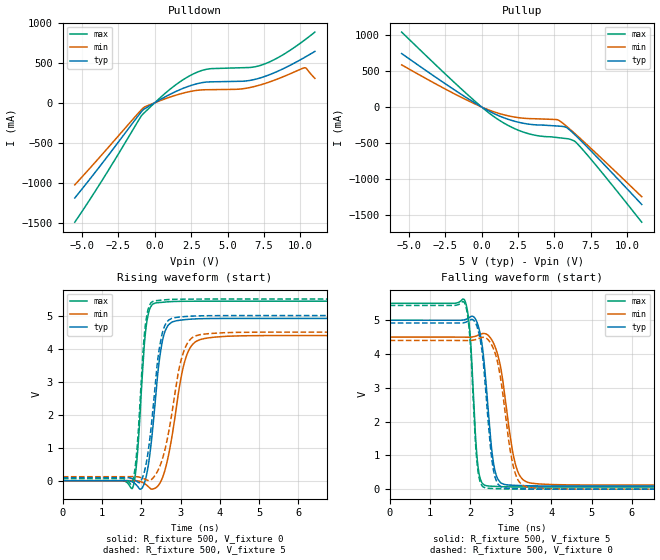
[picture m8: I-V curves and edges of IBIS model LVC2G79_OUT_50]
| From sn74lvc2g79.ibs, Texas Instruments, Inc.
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[Model]   LVC2G79_OUT_50
Model_type  Output
Vref =   0
Rref =   500
Cref =   50p
Vmeas =   2.5
| variable   typ   min   max
C_comp   8.95pF   5.46pF   12.36pF
| C_pullup   9.69pF   5.46pF   12.36pF
| C_pulldown   8.21pF   6.20pF   11.61pF
[Temperature Range]   40   100   -40
| Ambient temperature   25   85   -40
[Voltage range]   5   4.5   5.5
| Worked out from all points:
|   slope of the pulldown table from 0 to 0.75 V, typ, clamps not added: 9.73 ohm
|   slope of the pullup table from 0 to 0.75 V, typ, clamps not added: 9.16 ohm
|   rising waveform, R_fixture 500, V_fixture 0: 20-80 % time 258ps typ, 373ps min, 175ps max; typ from 0 V to 4.91 V
|   falling waveform, R_fixture 500, V_fixture 5: 20-80 % time 221ps typ, 319ps min, 148ps max; typ from 5 V to 0.091 V
|   rising waveform, R_fixture 500, V_fixture 5: 20-80 % time 265ps typ, 395ps min, 175ps max; typ from 0.091 V to 5 V
|   falling waveform, R_fixture 500, V_fixture 0: 20-80 % time 218ps typ, 313ps min, 147ps max; typ from 4.92 V to 0 V
[Pulldown]
| LVC2G79_OUT_50
|   Voltage   I(typ)   I(min)   I(max)
-5.5V     -1.19A     -1.026A    -1.493A
-3.615V   -756.5mA   -644.9mA   -968mA
-860mV    -99.61mA   -76.72mA   -149.6mA
1.145V    114mA      76.72mA    182.7mA
2.335V    206.5mA    136.8mA    330.4mA
3.39V     254.8mA    162mA      411mA
5.9V      268mA      171.6mA    436.9mA
6.79V     288.1mA    200.2mA    446mA
7.59V     330.6mA    241.7mA    487.6mA
8.82V     424.5mA    324.7mA    600.5mA
10.29V    565.4mA    436.9mA    781.9mA
11V       641.1mA    304.6mA    882.6mA
[Pullup]
| LVC2G79_OUT_50
|   Voltage   I(typ)   I(min)   I(max)
-5.5V     745.2mA    587.5mA    1.044A
-1.18V    147.6mA    112.6mA    211.7mA
1.04V     -109.2mA   -79.97mA   -161.6mA
2.045V    -185.4mA   -131.8mA   -280mA
3.05V     -232.7mA   -158.7mA   -361.3mA
3.945V    -250.5mA   -165.3mA   -402.5mA
5.295V    -265.8mA   -184.8mA   -427.6mA
5.83V     -285.1mA   -267.5mA   -440mA
6.335V    -372.8mA   -357.2mA   -470.5mA
6.54V     -412.8mA   -394.7mA   -503.8mA
8.12V     -739mA     -692.4mA   -876.8mA
11V       -1.358A    -1.25A     -1.605A
[Ramp]
| LVC2G79_OUT_50
| variable   typ   min   max
dV/dt_r   3.10/2.76E-10   2.79/4.06E-10   3.41/1.90E-10
dV/dt_f   3.02/2.32E-10   2.69/3.36E-10   3.34/1.55E-10
R_load = 500
[Rising Waveform]
| LVC2G79_OUT_50
R_fixture =   500
C_fixture =   0
L_fixture =   0
V_fixture =   0
V_fixture_min = 0
V_fixture_max = 0
|   Time   V(typ)   V(min)   V(max)
0s        185.3pV    4.77nV     2.097nV
1.78ns    -40.47mV   4.267mV    -217.7mV
1.895ns   -154.8mV   -1.104mV   706.8mV
2.125ns   123.6mV    -121.8mV   4.669V
2.375ns   2.639V     -210.8mV   5.385V
2.52ns    4.114V     31.46mV    5.4V
2.67ns    4.68V      634.9mV    5.416V
3.115ns   4.877V     3.642V     5.433V
3.605ns   4.908V     4.304V     5.435V
22.5ns    4.914V     4.397V     5.435V
[Falling Waveform]
| LVC2G79_OUT_50
R_fixture =   500
C_fixture =   0
L_fixture =   0
V_fixture =   5
V_fixture_min = 4.5
V_fixture_max = 5.5
|   Time   V(typ)   V(min)   V(max)
0s        5V         4.5V       5.5V
1.86ns    5.015V     4.498V     5.584V
1.99ns    5.093V     4.498V     4.616V
2.185ns   4.86V      4.553V     697.9mV
2.405ns   2.875V     4.583V     99.76mV
2.54ns    1.041V     4.396V     86.95mV
2.67ns    318.2mV    4.002V     78.52mV
3.105ns   113.5mV    781.3mV    66.24mV
3.5ns     99.06mV    178.3mV    63.91mV
22.5ns    91.35mV    120.7mV    62.83mV
[Rising Waveform]
| LVC2G79_OUT_50
R_fixture =   500
C_fixture =   0
L_fixture =   0
V_fixture =   5
V_fixture_min = 4.5
V_fixture_max = 5.5
|   Time   V(typ)   V(min)   V(max)
0s        91.33mV    120.7mV    62.82mV
1.765ns   63.77mV    124.3mV    -75.71mV
1.885ns   -17.21mV   121.4mV    880.2mV
2.105ns   400.1mV    39.54mV    4.708V
2.33ns    2.565V     126.3mV    5.444V
2.46ns    4V         398.4mV    5.461V
2.62ns    4.743V     1.023V     5.479V
3.055ns   4.965V     3.816V     5.497V
3.5ns     4.992V     4.422V     5.5V
22.5ns    5V         4.5V       5.5V
[Falling Waveform]
| LVC2G79_OUT_50
R_fixture =   500
C_fixture =   0
L_fixture =   0
V_fixture =   0
V_fixture_min = 0
V_fixture_max = 0
|   Time   V(typ)   V(min)   V(max)
0s        4.917V     4.401V     5.437V
1.855ns   4.93V      4.399V     5.514V
1.99ns    5.003V     4.399V     4.444V
2.175ns   4.768V     4.446V     656mV
2.37ns    3.048V     4.479V     38.69mV
2.525ns   929.1mV    4.272V     21.02mV
2.65ns    226.3mV    3.871V     14.06mV
3.065ns   18.23mV    659.6mV    3.351mV
3.42ns    7.426mV    55.16mV    1.203mV
22.5ns    16.82uV    25.77uV    12.87uV
